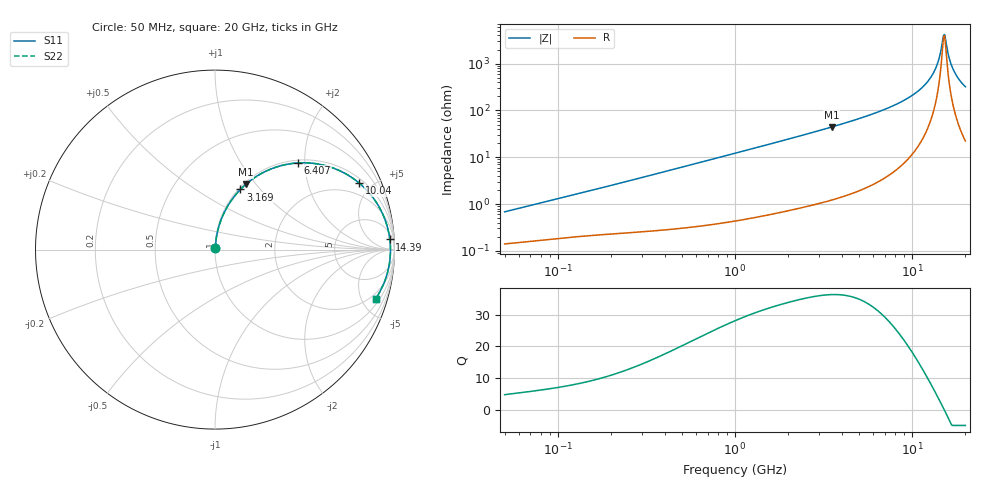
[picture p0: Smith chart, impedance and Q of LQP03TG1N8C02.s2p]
!Murata Part Number: LQP03TG1N8C02
!These Parameters are Measured in Series Mode Connection
!  o--[Z]--o
!Port1  Port2
!  o-------o
!Freq. Start=50[MHz] Stop=20[GHz], 401[Steps]
# Hz S RI R 50
!Freq.(Hz) S11(Real) S11(Imag) S21(Real) S21(Imag) S12(Real) S12(Imag) S22(Real) S22(Imag)
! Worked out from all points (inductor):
!   401 points, 50 MHz to 20 GHz, reference 50 ohm
!   read as one part in series: L = 2.09 nH near 51.52 MHz
!   highest Q = 36.4 at 3.519 GHz (marker M1), where L = 2 nH
!   self-resonance near 15.05 GHz
!   S11 on the Smith chart (normalised r, x): 50 MHz: 1.00, +0.01; 3.169 GHz: 1.02, +0.79; 6.407 GHz: 1.06, +1.85; 10.04 GHz: 1.23, +4.22; 14.39 GHz: 12, +29; 20 GHz: 1.44, -6.40
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5e7  0.00144 0.00663  0.9986 -0.00663  0.9986 -0.00663  0.00144 0.00663
1.364002e8  0.00233 0.0172  0.9977 -0.0172  0.9977 -0.0172  0.00233 0.0172
3.721004e8  0.00478 0.0453  0.9952 -0.0453  0.9952 -0.0453  0.00478 0.0453
1e9  0.0186 0.1187  0.9814 -0.1187  0.9814 -0.1187  0.0186 0.1187
2.728004e9  0.1084 0.2972  0.8916 -0.2972  0.8916 -0.2972  0.1084 0.2972
3.168813e9  0.1417 0.3352  0.8583 -0.3352  0.8583 -0.3352  0.1417 0.3352
3.519108e9  0.1706 0.3627  0.8294 -0.3627  0.8294 -0.3627  0.1706 0.3627
4.81993e9  0.2936 0.4415  0.7064 -0.4415  0.7064 -0.4415  0.2936 0.4415
6.406762e9  0.4618 0.4828  0.5382 -0.4828  0.5382 -0.4828  0.4618 0.4828
7.442007e9  0.5714 0.4772  0.4286 -0.4772  0.4286 -0.4772  0.5714 0.4772
1.004137e10  0.8038 0.3704  0.1962 -0.3704  0.1962 -0.3704  0.8038 0.3704
1.149051e10  0.8922 0.2732  0.1078 -0.2732  0.1078 -0.2732  0.8922 0.2732
1.276073e10  0.9428 0.1787  0.0572 -0.1787  0.0572 -0.1787  0.9428 0.1787
1.375312e10  0.966 0.1037  0.034 -0.1037  0.034 -0.1037  0.966 0.1037
1.438523e10  0.9741 0.0569  0.0259 -0.0569  0.0259 -0.0569  0.9741 0.0569
1.482269e10  0.977 0.0252  0.023 -0.0252  0.023 -0.0252  0.977 0.0252
1.527346e10  0.9777 -0.00669  0.0223 0.00669  0.0223 0.00669  0.9777 -0.00669
1.550395e10  0.9773 -0.0226  0.0227 0.0226  0.0227 0.0226  0.9773 -0.0226
1.646126e10  0.9705 -0.0859  0.0295 0.0859  0.0295 0.0859  0.9705 -0.0859
1.721783e10  0.9601 -0.1322  0.0399 0.1322  0.0399 0.1322  0.9601 -0.1322
1.855685e10  0.9332 -0.2058  0.0668 0.2058  0.0668 0.2058  0.9332 -0.2058
2e10  0.8958 -0.2728  0.1042 0.2728  0.1042 0.2728  0.8958 -0.2728
